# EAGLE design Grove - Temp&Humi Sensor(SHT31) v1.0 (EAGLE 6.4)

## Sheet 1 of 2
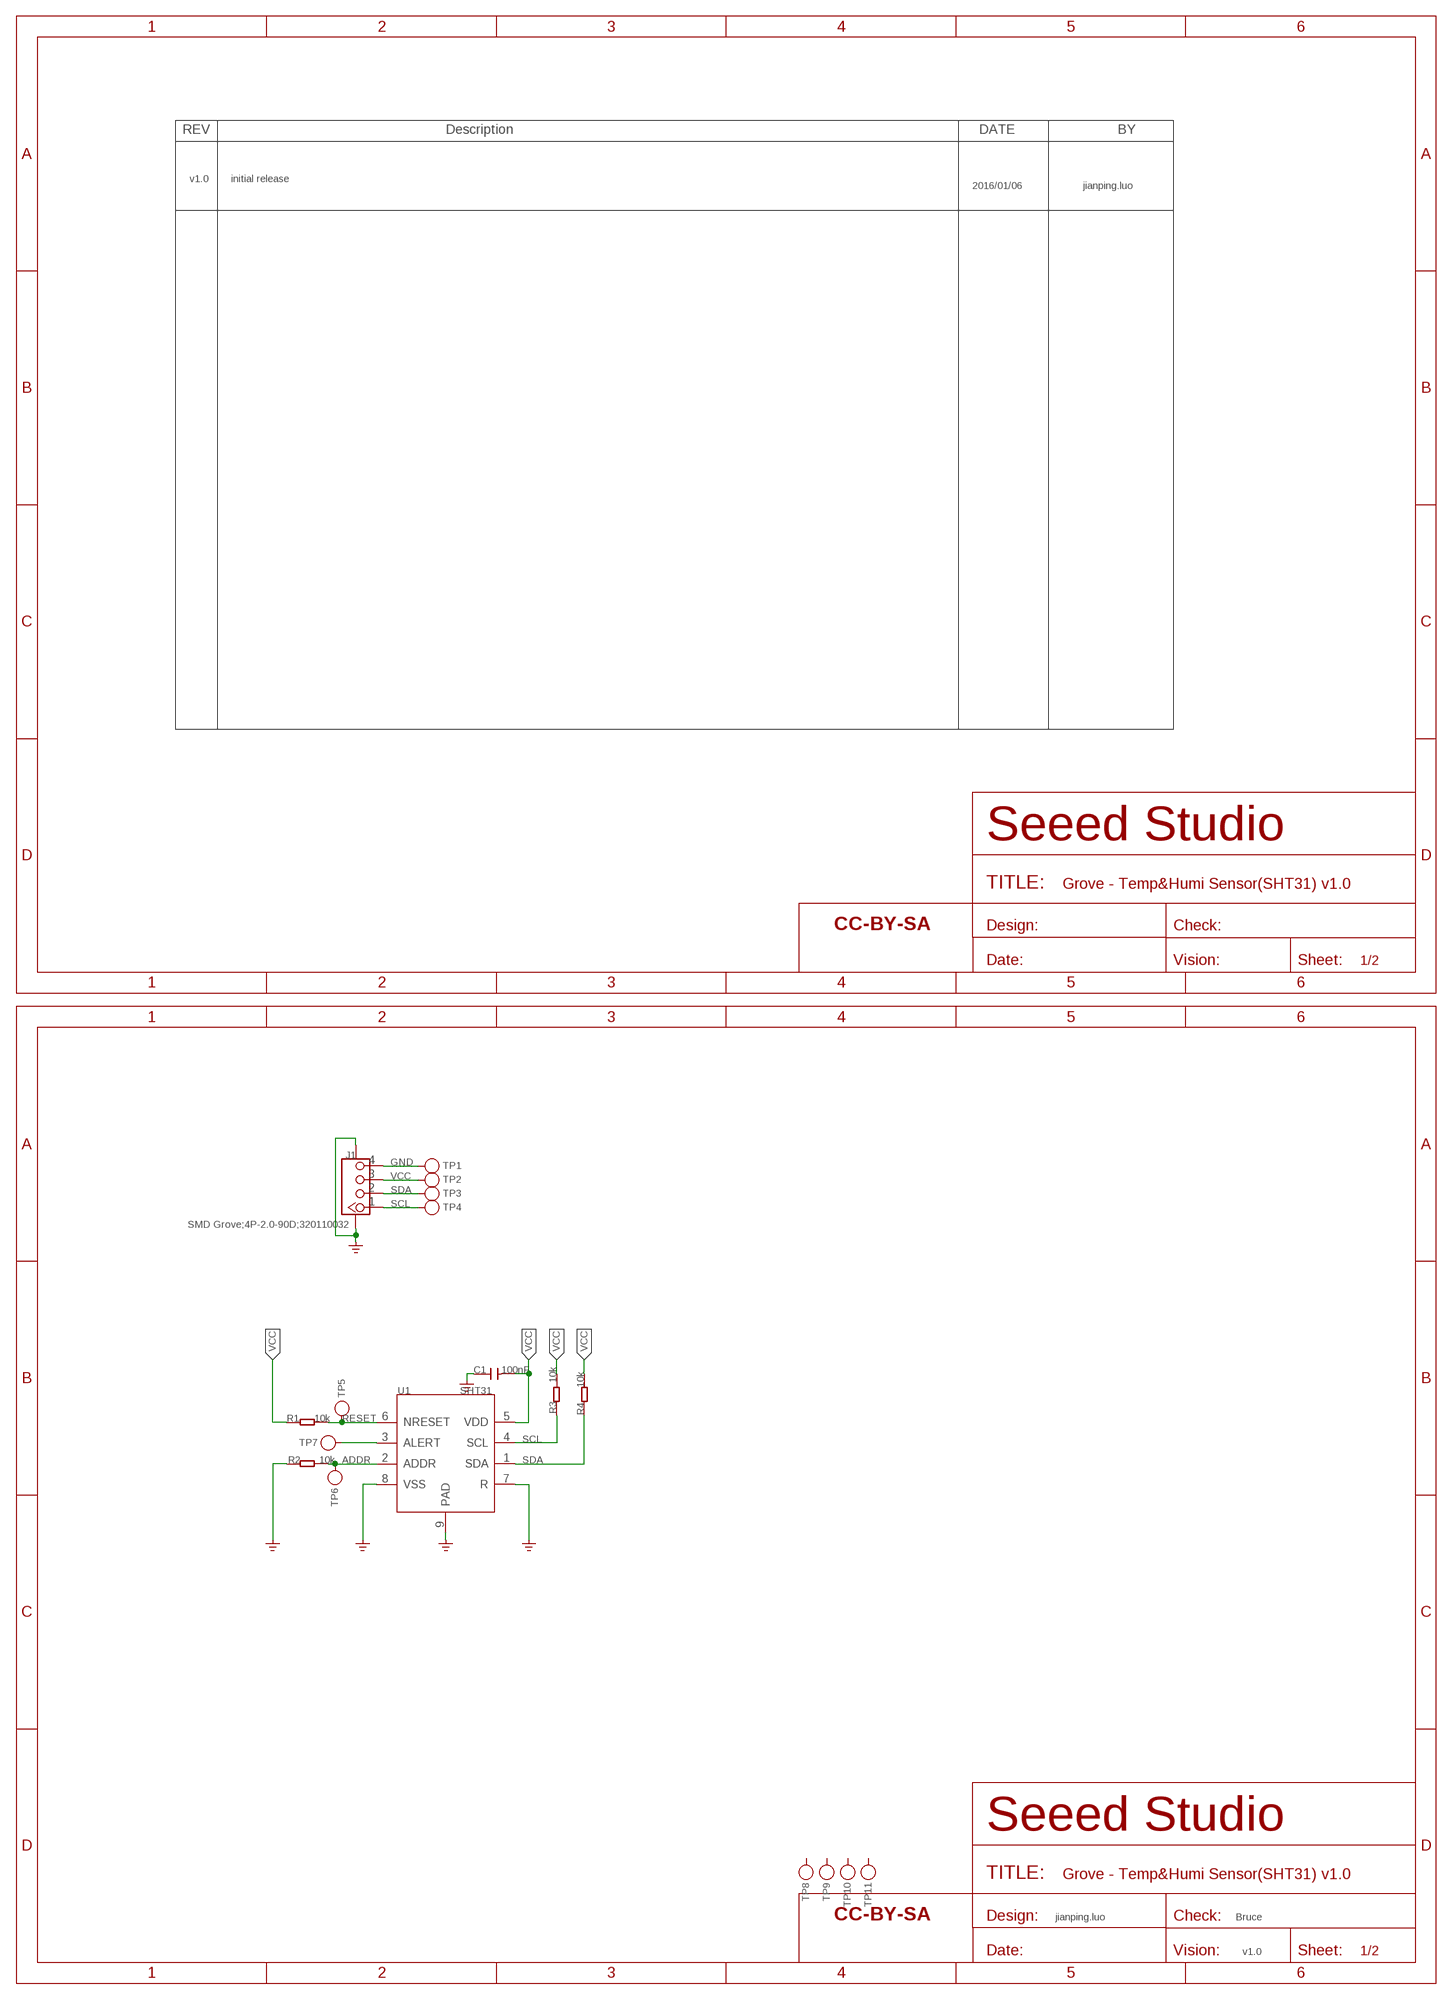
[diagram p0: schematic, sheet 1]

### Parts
C1  100nF  CAP-0603  [C0603]
FR1  SEEEDSTUDIO-OPEN-SCH-FRAME  [SEEEDSTUDIO-PCB-FRAME]
FR2  SEEEDSTUDIO-OPEN-SCH-FRAME  [SEEEDSTUDIO-PCB-FRAME]
J1  SMD Grove;4P-2.0-90D;320110032  GROVE-CONNECTOR-SMD'90D'  [HW4-SMD-2.0-90D]
R1  10k  RES-0603  [R0603]
R2  10k  RES-0603  [R0603]
R3  10k  RES-0603  [R0603]
R4  10k  RES-0603  [R0603]
TP1  TEST-POINT'4545'  [TP-D45MIL]
TP2  TEST-POINT'4545'  [TP-D45MIL]
TP3  TEST-POINT'4545'  [TP-D45MIL]
TP4  TEST-POINT'4545'  [TP-D45MIL]
TP5  TEST-POINT'4545'  [TP-D45MIL]
TP6  TEST-POINT'4545'  [TP-D45MIL]
TP7  TEST-POINT'4545'  [TP-D45MIL]
TP8  TEST-POINT'4545'  [TP-D45MIL]
TP9  TEST-POINT'4545'  [TP-D45MIL]
TP10  TEST-POINT'4545'  [TP-D45MIL]
TP11  TEST-POINT'4545'  [TP-D45MIL]
U1  SHT31  SENSOR-SHT3X-DIS  [DFN8-0.5-2.5X2.5MM]

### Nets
ADDR: R2.1 TP6.T U1.2(ADDR)
GND: C1.1 J1.4 J1.SS1 J1.SS2 R2.2 TP1.T U1.7(R) U1.8(VSS) U1.9(PAD) ; supply symbol labelled GND_POWER
N$1: TP7.T U1.3(ALERT)
RESET: R1.2 TP5.T U1.6(NRESET)
SCL: J1.1 R3.2 TP4.T U1.4(SCL)
SDA: J1.2 R4.1 TP3.T U1.1(SDA)
VCC: C1.2 J1.3 R1.1 R3.1 R4.2 TP2.T U1.5(VDD)
Unconnected: TP8.T TP9.T TP10.T TP11.T

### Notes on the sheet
- v1.0 | initial release
- 2016/01/06 | jianping.luo
- jianping.luo | Bruce
- v1.0

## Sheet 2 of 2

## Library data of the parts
C1 = Discrete-new:CAP: Ceramic Capacitors
FR1 FR2 = moudle-new:SEEEDSTUDIO-OPEN-SCH-FRAME
J1 = Connector-new:GROVE-CONNECTOR-SMD: 4P-SMD-2.0:320110030;4P-SMD-2.0-90D:320110032
R1-R4 = Discrete-new:RES
TP1-TP11 = Discrete-new:TEST-POINT; PARTNO: DNP
U1 = template:SENSOR-SHT3X-DIS

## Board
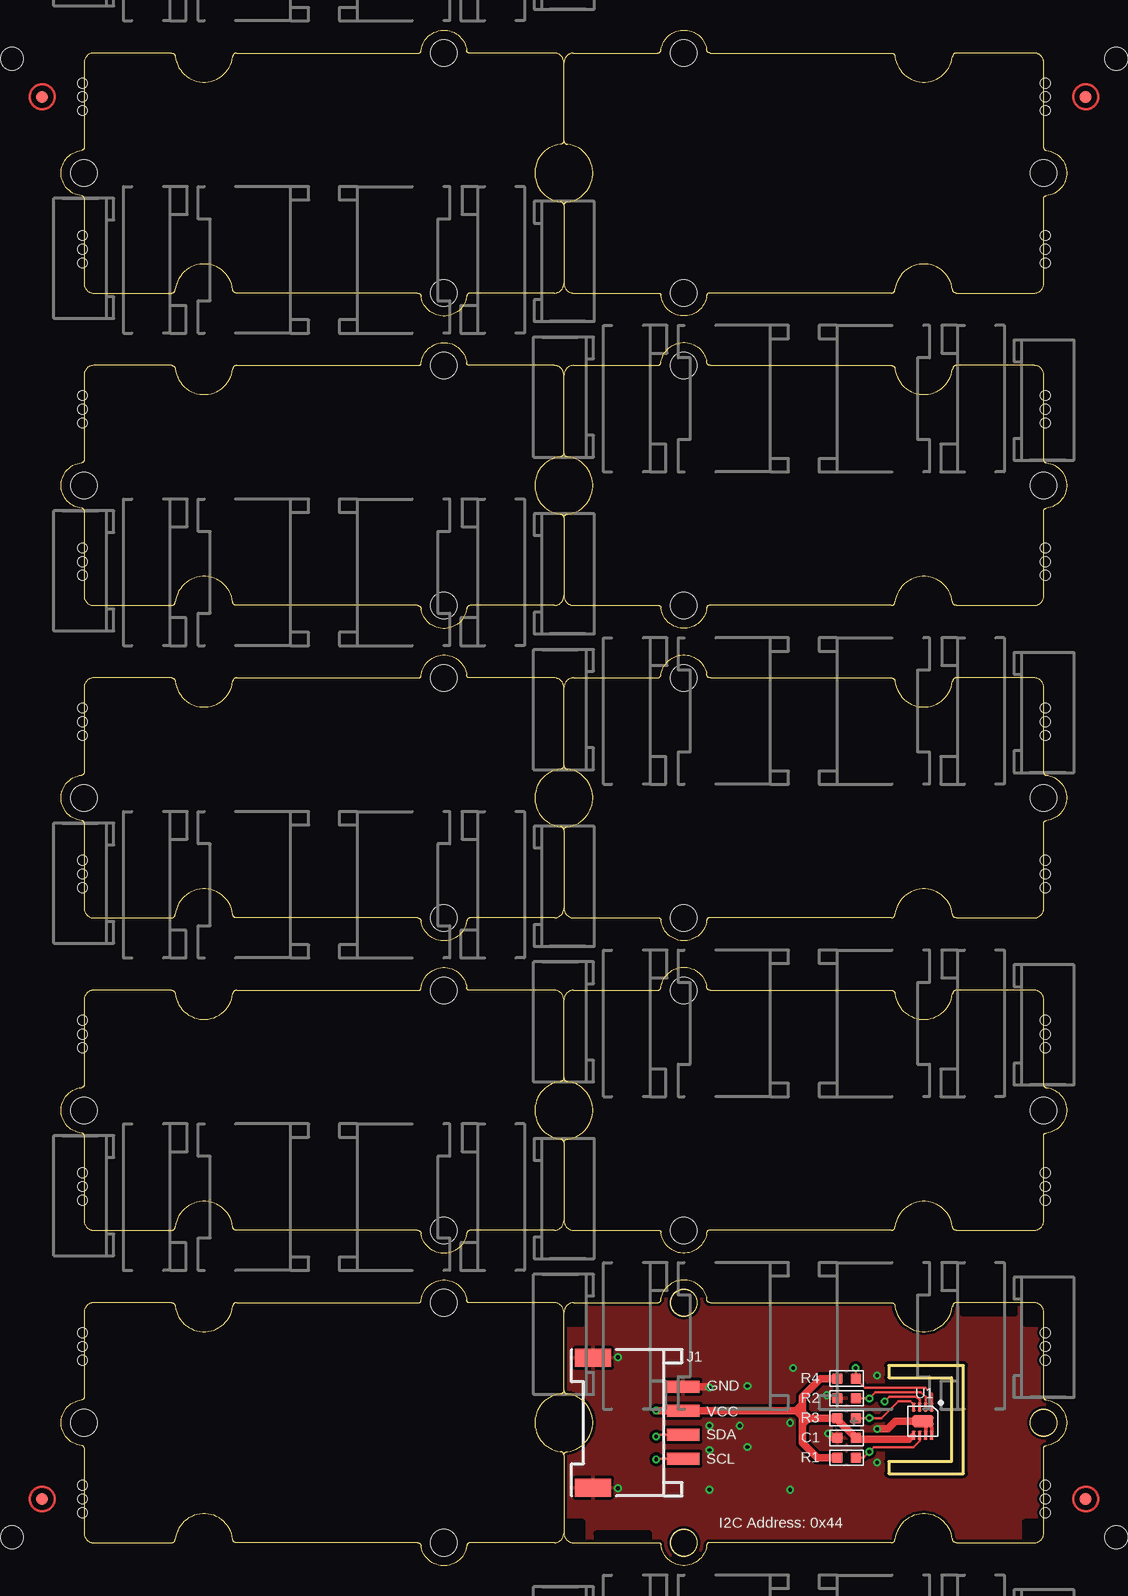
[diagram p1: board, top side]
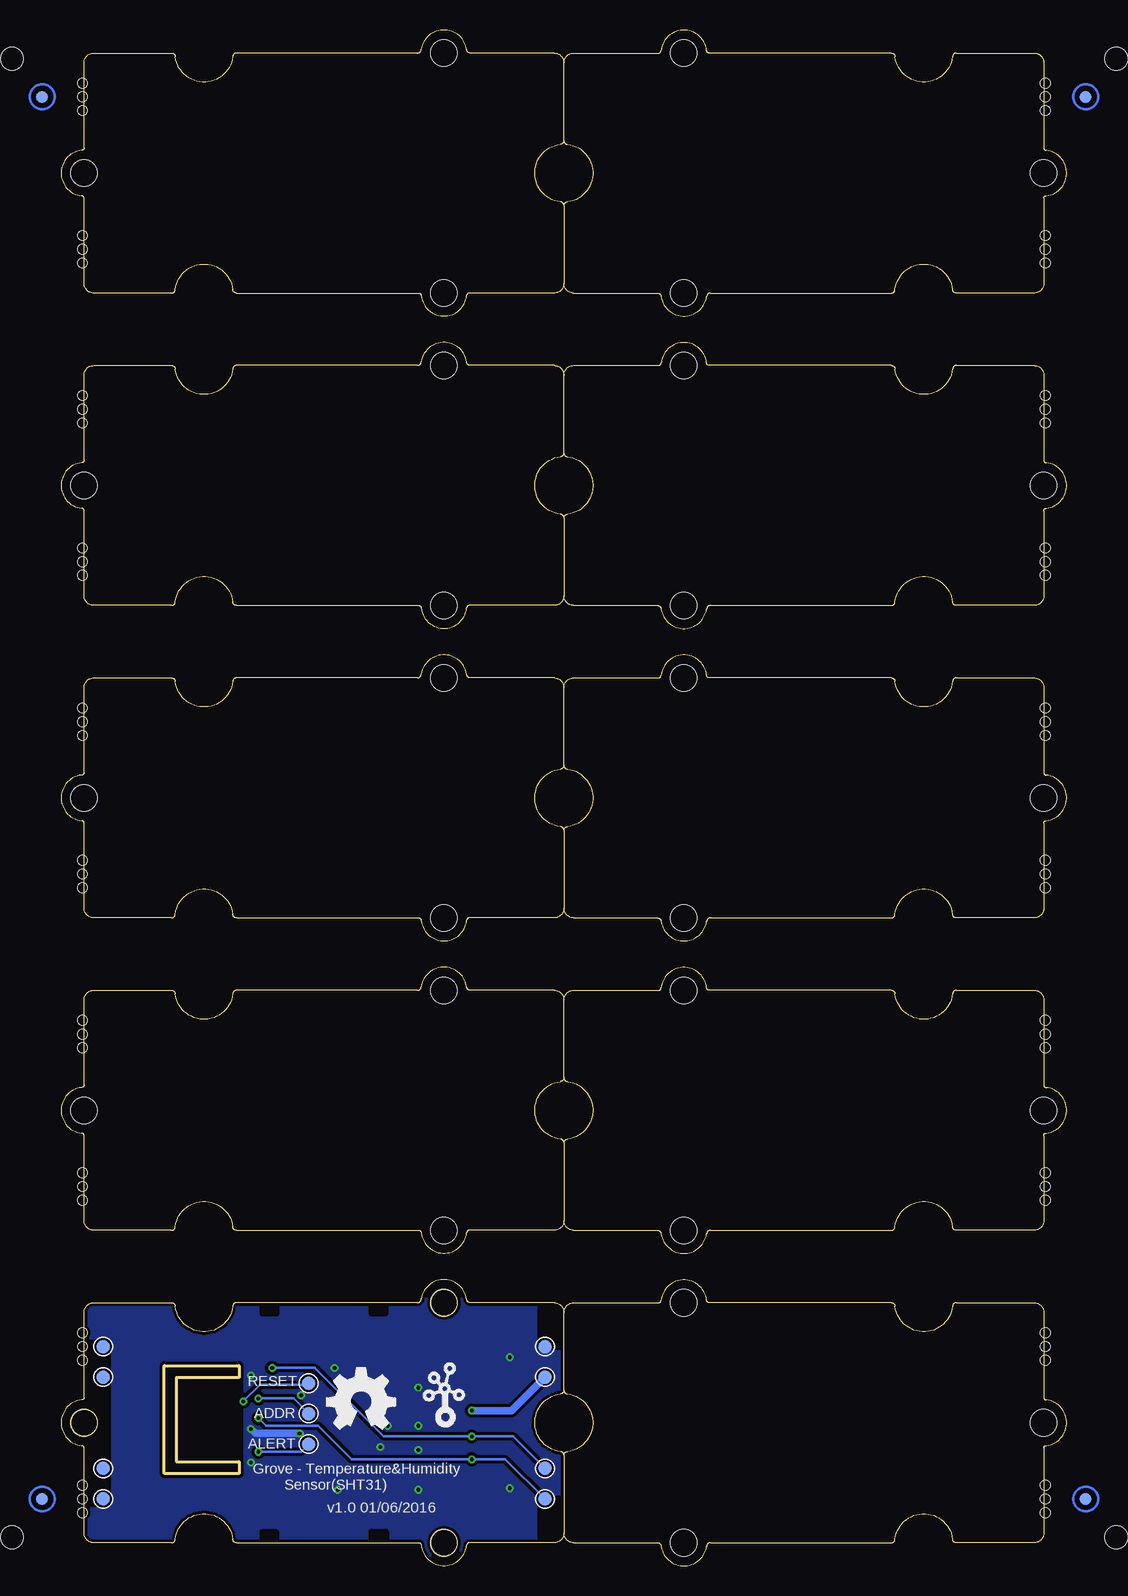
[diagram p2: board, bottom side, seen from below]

Size 83.82 x 127.98 mm. Coordinates in mm from the lower left corner, seen from the top.
Outline: 68.99,15.68 74.23,15.68 74.23,8.68 68.99,8.68 68.99,7.68 75.23,7.68 75.23,16.68 68.99,16.68 68.99,15.68
Copper layers (1*16): Top 0.035mm / dielectric 1.5mm / Bottom 0.035mm
Design rules "SeeedStudio_2layer_DRU_no_angle_20140221 *": minimum track width 6mil, minimum drill 12mil, track to track 6mil, track to pad 6mil, pad to pad 6mil, via to via 6mil, smd to smd 0mil, copper to edge 10mil, drill to drill 10mil, minimum pad ring 10mil, minimum via ring 6mil, stop-mask expansion 2mil, vias tented up to drill 25mil, thermal gap 10mil
Holes 0.8 mm at 82.04,4.43 82.04,6.71 82.04,5.57 82.04,17.13 82.04,19.41 82.04,18.27 82.04,30.46 82.04,32.75 82.04,31.61 82.04,43.16 82.04,45.45 82.04,44.31 82.04,56.5 82.04,58.78 82.04,57.64 82.04,69.2 82.04,71.48 82.04,70.34 82.04,82.53 82.04,84.82 82.04,83.68 82.04,95.23 82.04,97.52 82.04,96.38 82.04,108.57 82.04,110.85 82.04,109.71 82.04,121.27 82.04,123.55 82.04,122.41 1.78,6.71 1.78,4.43 1.78,5.57 1.78,19.41 1.78,17.13 1.78,18.27 1.78,32.75 1.78,30.46 1.78,31.61 1.78,45.45 1.78,43.16 1.78,44.31 1.78,58.78 1.78,56.5 1.78,57.64 1.78,71.48 1.78,69.2 1.78,70.34 1.78,84.82 1.78,82.53 1.78,83.68 1.78,97.52 1.78,95.23 1.78,96.38 1.78,110.85 1.78,108.57 1.78,109.71 1.78,123.55 1.78,121.27 1.78,122.41
Holes 1.91 mm at 87.95,125.59 -4.13,125.59 -4.13,2.4 87.95,2.4
tRestrict: area 68.9,7.6 to 75.2,16.7
bRestrict: area 68.9,7.6 to 75.2,16.7

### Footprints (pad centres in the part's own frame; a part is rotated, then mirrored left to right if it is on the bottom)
C0603 = smd 0.889 x 0.889: 1 0,0.762; 2 0,-0.762
HW4-SMD-2.0-90D = smd 1.01 x 2.74: 1 -3,-0.1; 2 -1,-0.1; 3 1,-0.1; 4 3,-0.1 | smd 1.5 x 3: SS1 -5.4,7.4; SS2 5.4,7.4
ROUND-MARK-1.0 = smd 1.016 x 1.016: P$1 0,0
R0603 = smd 0.889 x 0.889: 1 0,0.762; 2 0,-0.762
TP-D45MIL = smd 1.143 x 1.143: T 0,0
DFN8-0.5-2.5X2.5MM = smd 0.75 x 0.3: 1 -1.175,0.75; 2 -1.175,0.25; 3 -1.175,-0.25; 4 -1.175,-0.75; 5 1.175,-0.75; 6 1.175,-0.25; 7 1.175,0.25; 8 1.175,0.75 | smd 1 x 1.8: 9 0,0
GROVE-TEST-PLATFORM = hole 2.2: -10,-10; -10,10; 20,0
GROVE-1*2-TEST-PLATFORM = hole 2.2: 10.635,10; 10.635,-10; -19.365,0

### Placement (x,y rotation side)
C1  65.47,10.65 90 top
FR1  not placed on the board
FR2  not placed on the board
J1  51.75,11.92 90 top
P1  [ROUND-MARK-1.0]  85.41,122.41 180 top
P2  [ROUND-MARK-1.0]  -1.59,122.41 180 top
P3  [ROUND-MARK-1.0]  85.41,5.57 180 top
P4  [ROUND-MARK-1.0]  -1.59,5.57 180 top
P5  [ROUND-MARK-1.0]  85.41,122.41 180 bottom
P6  [ROUND-MARK-1.0]  -1.59,122.41 180 bottom
P7  [ROUND-MARK-1.0]  -1.59,5.57 180 bottom
P8  [ROUND-MARK-1.0]  85.41,5.57 180 bottom
R1  65.47,9 90 top
R2  65.47,13.95 270 top
R3  65.47,12.3 90 top
R4  65.47,15.6 270 top
TP1  43.5,18.27 0 bottom
TP2  43.5,15.73 0 bottom
TP3  43.5,8.11 0 bottom
TP4  43.5,5.57 0 bottom
TP5  63.18,10.14 180 bottom
TP6  63.18,12.68 180 bottom
TP7  63.18,15.22 180 bottom
TP8  80.33,5.57 180 bottom
TP9  80.33,8.11 180 bottom
TP10  80.33,15.73 180 bottom
TP11  80.33,18.27 180 bottom
U1  71.82,12.05 270 top
U2  [GROVE-TEST-PLATFORM]  21.91,90.03 180 top
U3  [GROVE-TEST-PLATFORM]  61.91,90.03 0 top
U4  [GROVE-TEST-PLATFORM]  21.91,63.99 180 top
U5  [GROVE-TEST-PLATFORM]  61.91,63.99 0 top
U6  [GROVE-TEST-PLATFORM]  21.91,37.96 180 top
U7  [GROVE-TEST-PLATFORM]  61.91,37.96 0 top
U8  [GROVE-TEST-PLATFORM]  61.91,11.92 0 top
U9  [GROVE-TEST-PLATFORM]  21.91,11.92 180 top
U10  [GROVE-TEST-PLATFORM]  21.91,116.06 180 top
U11  [GROVE-TEST-PLATFORM]  61.91,116.06 0 top
U$7  [GROVE-1*2-TEST-PLATFORM]  62.55,11.92 180 top
U$8  TWIGLOGOTWIGLOGO_SMALL  [TWIGLOGO_SMALL]  54.04,11.41 0 bottom
U$9  [OSHW_FILLX200_NOTEXT]  61.66,11.41 0 bottom

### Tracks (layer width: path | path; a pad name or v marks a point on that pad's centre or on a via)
ADDR  (via drill 0.3 pad 0.64)
  Top 0.203: U1.2 72.07,14.08 71.69,14.46 67.88,14.46 v67.37,13.95 R2.1
  Bottom 0.203: v67.37,13.95 64.45,13.95 TP6.T
GND  (via drill 0.3 pad 0.64)
  Top 0.305: U1.7 72.07,11.8 | 72.07,11.8 U1.9 | U1.8 72.57,11.55 72.33,11.79 72.07,11.79 72.07,11.8
  Top 0.61: J1.4 53.96,14.92 v54.04,14.84 | C1.1 64.33,10.65 v63.95,11.03 | U1.9 69.53,12.05 68.9,11.41 v68.01,11.41
  Bottom 0.61: v63.95,11.03 67.63,11.03 v68.01,11.41
  other vias: 63.82,14.21 68.01,8.62 68.01,15.86 46.42,6.46 60.77,11.92 57.21,9.89 54.04,9.64 54.04,11.67 56.58,11.67 57.21,14.97 46.42,17.38 54.04,6.33 60.77,6.33 61.02,16.49
  pour Bottom (isolate 0.254): 41.34,22.21 81.98,22.21 81.98,0.62 41.34,0.62
  pour Top (isolate 0.254): 41.34,22.21 81.98,22.21 81.98,0.62 41.34,0.62
N$1  (via drill 0.3 pad 0.64)
  Top 0.203: U1.3 71.57,13.82 71.31,14.08 69.03,14.08 v68.64,13.7
  Bottom 0.203: TP7.T 63.31,15.1 67.25,15.1 v68.64,13.7
RESET  (via drill 0.3 pad 0.64)
  Top 0.203: R1.2 66.87,9 v67.37,9.51 67.76,9.89 71.06,9.89 71.57,10.4 U1.6
  Bottom 0.203: v67.37,9.51 63.82,9.51 TP5.T
SCL  (via drill 0.3 pad 0.64)
  Top 0.203: U1.4 71.07,13.43 70.8,13.7 69.79,13.7 68.39,12.3 v67.37,12.3 R3.2 | J1.1 49.64,8.92 v49.59,8.87
  Bottom 0.203: TP4.T 46.8,8.87 v49.59,8.87 59.63,8.87 62.42,11.67 66.74,11.67 v67.37,12.3
SDA  (via drill 0.3 pad 0.64)
  Top 0.203: U1.1 72.57,14.33 72.06,14.84 66.99,14.84 R4.1 v66.23,16.49 | J1.2 49.74,10.92 v49.59,10.78
  Bottom 0.203: TP3.T 46.17,10.78 v49.59,10.78 56.96,10.78 62.68,16.49 v66.23,16.49
VCC  (via drill 0.3 pad 0.64)
  Top 0.305: 70.87,10.52 71.07,10.73 U1.5 71.03,10.87 70.8,10.65 70.68,10.65 | 70.87,10.52 70.61,10.52 | 70.87,10.52 70.74,10.4 70.49,10.4 | 70.36,10.65 70.68,10.65 | 70.68,10.65 71.06,11.03
  Top 0.61: 70.61,10.52 66.36,10.52 C1.2 64.71,12.18 R3.1 62.29,12.3 | 61.26,12.92 J1.3 49.61,12.92 v49.59,12.94 | 61.29,12.92 61.77,12.92 61.79,12.94 | 61.79,13.45 61.79,14.08 63.31,15.6 R4.2 | 61.79,13.45 61.79,12.94 | 61.79,12.94 61.79,12.81 | 61.79,12.81 61.79,12.43 | 61.79,12.43 61.79,11.79 | 61.79,11.79 61.79,10.27 63.06,9 R1.1 | 61.26,12.92 61.79,13.45 | 61.26,12.92 61.29,12.92 | 61.29,12.92 61.79,12.43 | 62.29,12.3 61.91,12.3 61.79,12.43 | 62.29,12.3 61.79,12.81 | 62.29,12.3 61.79,11.79
  Bottom 0.61: v49.59,12.94 46.29,12.94 TP2.T

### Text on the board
tPlace: GND | VCC | SDA | SCL | I2C Address: 0x44
bPlace: RESET | ADDR | ALERT | Grove - Temperature&Humidity / Sensor(SHT31) | v1.0 01/06/2016

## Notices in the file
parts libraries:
moudle-new: This work is licensed under the Creative Commons Attribution 4.0 International License.
To view a copy of this license,visit:
http://creativecommons.org/licenses/by-sa/4.0
moudle-new: CC-BY-SA
